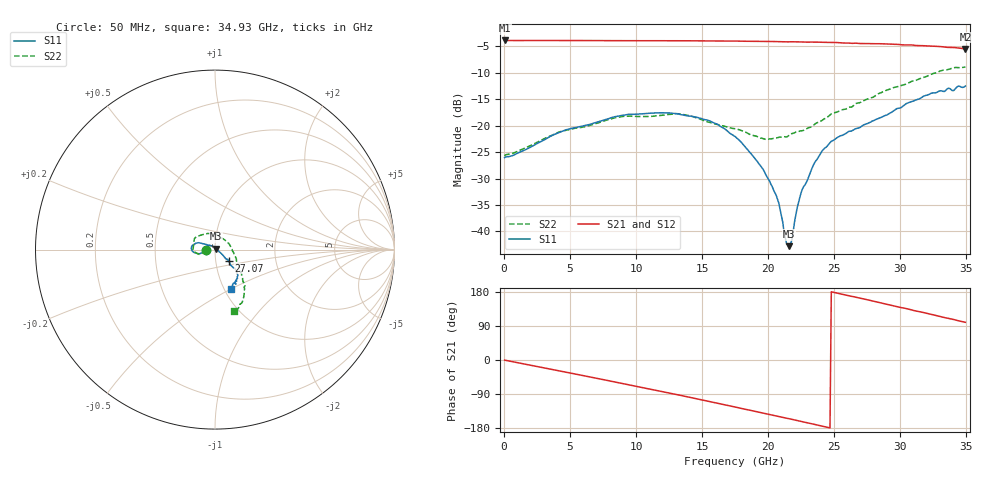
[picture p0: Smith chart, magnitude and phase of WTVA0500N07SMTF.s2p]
! 50 ohm 2-Port S-parameters measured by Modelithics Inc support@modelithics.com  Tampa, FL USA 813-866-6335 (February 2024)
! Smiths Interconnect,  5dB P/N: WTVA0500N07SMTF, Temperature: 75 C
! Board: 10 mil Rogers 4350B, Mounting Pad Dimensions: Length: 15 mils, Width: 25 mils, Gap: 40 mils.
# Hz S RI R 50
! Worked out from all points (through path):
!   352 points, 50 MHz to 34.93 GHz, reference 50 ohm
!   highest |S21| = -3.93 dB at 100 MHz (marker M1); lowest = -5.5 dB at 34.93 GHz (marker M2)
!   group delay of S21, straight-line fit = 20.7 ps
!   lowest |S11| = -42.8 dB at 21.59 GHz (marker M3), VSWR 1.01, Z = 50.5 + j0.502 ohm
!   |S11| at or under -10 dB: start of sweep to end of sweep
!   |S22| runs from -25.7 to -8.9 dB; largest |S21 - S12| = 0.0078
!   S11 on the Smith chart (normalised r, x): 50 MHz: 0.91, +0.00; 27.07 GHz: 1.16, -0.14; 34.93 GHz: 1.07, -0.50
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5e7  -0.0498 0.000161  0.6361 -0.00344  0.6356 -0.0033  -0.0517 -0.00156
1e8  -0.0504 -0.000863  0.6364 -0.00776  0.6357 -0.00785  -0.0528 -0.0016
2.986e9  -0.0705 -0.0169  0.596 -0.2213  0.5951 -0.2219  -0.0719 -0.0206
5.8715e9  -0.0958 -0.0227  0.484 -0.4111  0.4835 -0.4109  -0.0931 -0.024
8.8565e9  -0.1237 -0.0113  0.3058 -0.5544  0.304 -0.5545  -0.121 -0.00574
1.1742e10  -0.1318 0.00763  0.0924 -0.6251  0.0909 -0.6246  -0.1188 0.0369
1.3334e10  -0.1252 0.0239  -0.0342 -0.6311  -0.0358 -0.6303  -0.1111 0.0653
1.5523e10  -0.1055 0.036  -0.2086 -0.5945  -0.2109 -0.5928  -0.0674 0.0838
1.7513e10  -0.0711 0.0336  -0.3531 -0.5196  -0.3535 -0.5184  -0.0227 0.0902
2.01e10  -0.0207 0.0217  -0.5021 -0.3682  -0.502 -0.3672  0.0442 0.0605
2.07965e10  -0.00696 0.0173  -0.533 -0.3179  -0.5327 -0.3169  0.0588 0.0503
2.13935e10  0.00305 0.00694  -0.5526 -0.274  -0.5525 -0.2728  0.0672 0.0397
2.15925e10  0.0053 0.00497  -0.56 -0.2613  -0.5601 -0.2593  0.0719 0.0376
2.17915e10  0.00793 0.00251  -0.5672 -0.245  -0.5672 -0.2436  0.0773 0.0325
2.21895e10  0.0163 -0.00306  -0.5791 -0.2139  -0.5791 -0.2117  0.0845 0.0221
2.2488e10  0.0214 -0.00875  -0.5866 -0.1902  -0.5866 -0.1878  0.0879 0.0153
2.33835e10  0.0352 -0.0218  -0.603 -0.1175  -0.6025 -0.1172  0.0989 -0.0101
2.47765e10  0.0555 -0.0444  -0.6099 0.000181  -0.6093 0.00169  0.1185 -0.0504
2.7065e10  0.0771 -0.0611  -0.5673 0.1803  -0.5658 0.1825  0.135 -0.0995
2.91545e10  0.0926 -0.0907  -0.4872 0.3303  -0.4832 0.3347  0.1534 -0.1574
3.27365e10  0.1184 -0.1674  -0.2552 0.4992  -0.2524 0.4998  0.1554 -0.2739
3.49255e10  0.0874 -0.2193  -0.0881 0.5224  -0.0873 0.5215  0.1073 -0.3415
